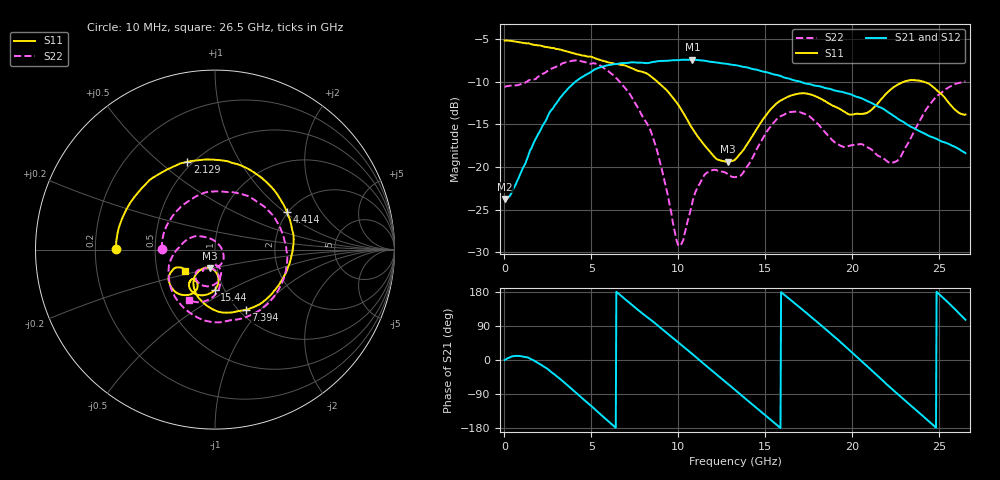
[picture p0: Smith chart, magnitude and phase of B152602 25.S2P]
!  2-Port S-parameters saved by WinCal
! VAR MeasName=S-Parameters (CALIBRATED_DATA) read from VNA (N5242A)
! VAR MeasDate=2016-1-5 16:28:50
! VAR NAME=B152602 25
! VAR FILENAME=B152602 25.S2P
! VAR DATE=2016-1-5 16:28:50
! VAR PHYS_PORTS=1,2
# Hz S DB R 50
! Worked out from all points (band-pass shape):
!   801 points, 10 MHz to 26.5 GHz, reference 50 ohm
!   highest |S21| = -7.40 dB at 10.8 GHz (marker M1); lowest = -23.8 dB at 43.11 MHz (marker M2)
!   |S21| within 3 dB of the highest: 3.862 GHz to 17.74 GHz (13.88 GHz wide, 128 % of centre)
!   lowest |S11| = -19.4 dB at 12.82 GHz (marker M3), VSWR 1.24, Z = 46.4 - j9.75 ohm
!   |S11| at or under -10 dB: 8.797 GHz to 22.97 GHz (14.17 GHz wide, 89.2 % of centre); 24.1 GHz to end of sweep
!   |S22| runs from -29.3 to -7.5 dB; largest |S21 - S12| = 0.0033
!   S11 on the Smith chart (normalised r, x): 10 MHz: 0.29, +0.00; 2.129 GHz: 0.47, +0.62; 4.414 GHz: 1.96, +1.05; 7.394 GHz: 1.07, -0.84; 15.44 GHz: 0.90, -0.43; 26.5 GHz: 0.70, -0.17
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1e7  -5.16 179.6  -23.72 -0.1  -23.73 0.3  -10.60 179.6
4.31125e7  -5.16 178.5  -23.77 0.6  -23.76 0.7  -10.59 177.8
1.301388e9  -5.51 135.8  -19.10 6.8  -19.10 6.8  -10.02 105.7
2.1292e9  -5.79 107.4  -15.42 -13.0  -15.42 -13.0  -9.11 58.7
3.288138e9  -6.27 67.0  -11.67 -53.5  -11.68 -53.5  -7.88 -3.6
4.413962e9  -6.88 28.0  -9.51 -98.7  -9.52 -98.6  -7.60 -58.7
4.447075e9  -6.91 26.9  -9.47 -100.0  -9.47 -100.0  -7.61 -60.1
6.036475e9  -7.75 -24.5  -8.04 -164.4  -8.03 -164.3  -8.88 -122.5
7.394088e9  -8.47 -62.9  -7.73 143.0  -7.73 143.1  -12.08 -168.3
8.851038e9  -10.11 -99.5  -7.58 89.7  -7.54 89.7  -18.69 139.8
1.000998e10  -12.76 -121.4  -7.47 46.2  -7.44 46.2  -29.20 49.3
1.080468e10  -15.52 -127.6  -7.40 15.6  -7.39 15.5  -24.14 -38.5
1.159938e10  -17.70 -123.8  -7.57 -15.4  -7.55 -15.5  -20.73 -71.9
1.282454e10  -19.37 -104.7  -7.91 -62.3  -7.92 -62.2  -20.82 -91.3
1.3255e10  -19.14 -95.6  -8.06 -78.7  -8.04 -78.7  -21.20 -88.3
1.421526e10  -16.49 -83.5  -8.49 -116.0  -8.44 -115.9  -19.14 -75.4
1.544042e10  -12.95 -90.3  -9.11 -162.9  -9.06 -162.9  -14.88 -85.1
1.769208e10  -11.54 -120.3  -10.37 111.2  -10.33 111.3  -14.34 -124.4
1.997684e10  -13.86 -125.0  -11.54 20.2  -11.54 20.1  -17.46 -119.6
2.209604e10  -11.10 -117.7  -13.63 -69.0  -13.57 -69.2  -19.46 -108.3
2.428146e10  -10.12 -145.7  -16.23 -157.0  -16.20 -157.3  -13.14 -84.0
2.65e10  -13.85 -144.6  -18.38 106.2  -18.37 106.1  -9.99 -116.9
